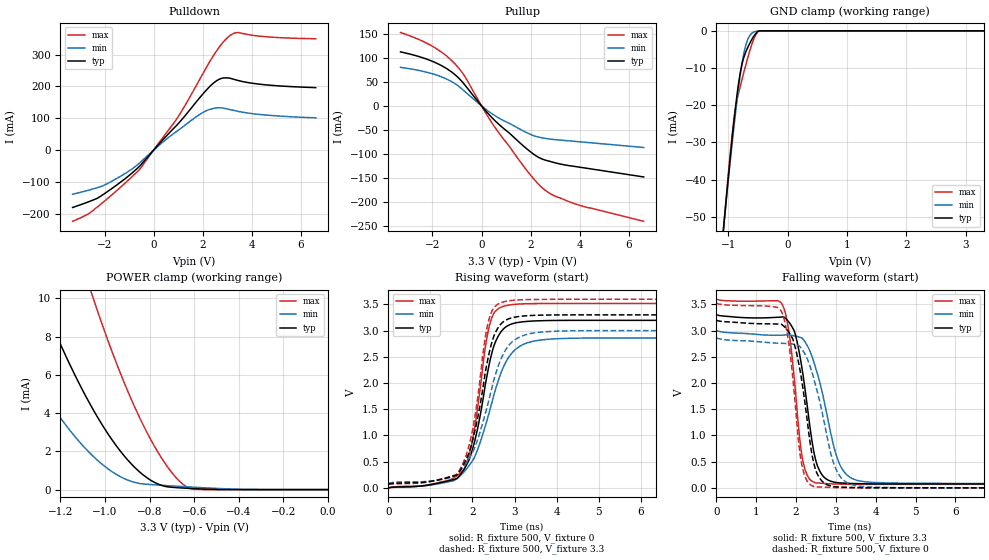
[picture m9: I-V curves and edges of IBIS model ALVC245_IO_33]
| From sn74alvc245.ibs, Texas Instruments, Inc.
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[Model]   ALVC245_IO_33
Model_type  I/O
Vinl=0.8
Vinh=2.0
Enable   Active-Low
Vref =   0
Rref =   500
Cref =   50p
Vmeas =   1.5
| variable   typ   min   max
C_comp   8.35pF   7.81pF   9.09pF
| C_pullup   10.69pF   8.03pF   12.78pF
| C_pulldown   13.57pF   8.50pF   20.76pF
| C_tri-state   8.35pF   7.81pF   9.09pF
[Temperature Range]   40   100   -40
| Ambient temperature   25   85   -40
[Voltage range]   3.3   3   3.6
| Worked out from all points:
|   slope of the pulldown table from 0 to 0.495 V, typ, clamps not added: 11.7 ohm
|   slope of the pullup table from 0 to 0.495 V, typ, clamps not added: 17.6 ohm
|   GND clamp passes 1 mA (typ) near -0.55 V on its own axis
|   POWER clamp passes 1 mA (typ) near -0.85 V on its own axis
|   rising waveform, R_fixture 500, V_fixture 0: 20-80 % time 492ps typ, 686ps min, 390ps max; typ from 0 V to 3.2 V
|   falling waveform, R_fixture 500, V_fixture 3.3: 20-80 % time 376ps typ, 552ps min, 281ps max; typ from 3.3 V to 0.073 V
|   rising waveform, R_fixture 500, V_fixture 3.3: 20-80 % time 484ps typ, 664ps min, 403ps max; typ from 0.073 V to 3.3 V
|   falling waveform, R_fixture 500, V_fixture 0: 20-80 % time 382ps typ, 537ps min, 285ps max; typ from 3.2 V to 0 V
[GND Clamp]
| ALVC245_IO_33
|   Voltage   I(typ)   I(min)   I(max)
-3.3V     -490.9mA   -462.1mA   -523.9mA
-1.08V    -53.52mA   -53.36mA   -53.54mA
-1.06V    -50.03mA   -50.1mA    -49.79mA
-965mV    -34.02mA   -35.1mA    -32.92mA
-910mV    -25.42mA   -26.89mA   -24.65mA
-865mV    -19.02mA   -20.55mA   -19.71mA
-810mV    -12.51mA   -13.51mA   -15.72mA
-765mV    -8.79mA    -8.615mA   -12.94mA
-705mV    -5.752mA   -3.933mA   -9.277mA
-575mV    -1.611mA   -356.2uA   -2.46mA
-475mV    -22.44uA   -72.78uA   -18.11uA
3.3V      121pA      1.473uA    20.6pA
[POWER Clamp]
| ALVC245_IO_33
|   Voltage   I(typ)   I(min)   I(max)
-3.3V     99.98mA    69.88mA    142.9mA
-1.515V   17.25mA    10.07mA    30.01mA
-1.39V    13.1mA     7.28mA     23.94mA
-1.295V   10.22mA    5.398mA    19.63mA
-1.175V   6.968mA    3.359mA    14.59mA
-1.055V   4.22mA     1.764mA    10.08mA
-950mV    2.303mA    801.1uA    6.651mA
-845mV    925.8uA    321uA      3.771mA
-745mV    216.5uA    225uA      1.628mA
-655mV    85.43uA    160.6uA    324.5uA
-600mV    50.05uA    123.9uA    17.12uA
-48.03fV  121pA      541.2pA    23.35pA
[Pulldown]
| ALVC245_IO_33
|   Voltage   I(typ)   I(min)   I(max)
-3.3V     -180.2mA   -138.9mA   -223.6mA
-2.675V   -163.1mA   -126.5mA   -201.3mA
-2.27V    -150.3mA   -117.4mA   -177.2mA
-1.355V   -101.2mA   -82.56mA   -117mA
-550mV    -48.67mA   -38.97mA   -58.59mA
955mV     79.19mA    59.82mA    99.87mA
1.96V     172.1mA    116.1mA    233.8mA
2.59V     219mA      132.6mA    314.7mA
3.1V      225.7mA    127.4mA    359.2mA
3.435V    218.6mA    121.6mA    369mA
4.63V     204.5mA    109.7mA    355.6mA
6.6V      196.1mA    101.2mA    349.6mA
[Pullup]
| ALVC245_IO_33
|   Voltage   I(typ)   I(min)   I(max)
-3.3V     112.1mA    79.99mA    152.2mA
-1.985V   92.16mA    66.47mA    123.3mA
-1.48V    79.23mA    57.07mA    105.8mA
-1.05V    63.39mA    45.04mA    85.45mA
-665mV    42.48mA    29.16mA    59.86mA
130mV     -7.91mA    -5.33mA    -11.38mA
615mV     -34.03mA   -22.47mA   -49.68mA
1.98V     -94.75mA   -58.81mA   -142.7mA
2.575V    -112.2mA   -67.23mA   -174.4mA
2.995V    -118.1mA   -69.95mA   -187.3mA
3.94V     -126.8mA   -74.19mA   -205.4mA
6.6V      -147.4mA   -86.26mA   -239.4mA
[Ramp]
| ALVC245_IO_33
| variable   typ   min   max
dV/dt_r   1.92/5.03E-10   1.72/6.88E-10   2.11/3.98E-10
dV/dt_f   1.94/4.01E-10   1.75/5.64E-10   2.12/2.84E-10
R_load = 500
[Rising Waveform]
| ALVC245_IO_33
R_fixture =   500
C_fixture =   0
L_fixture =   0
V_fixture =   0
V_fixture_min = 0
V_fixture_max = 0
|   Time   V(typ)   V(min)   V(max)
0s        400.7pV    3.194nV    69.15pV
1.43ns    134mV      115.4mV    143.4mV
1.8ns     356.3mV    305.9mV    346.1mV
2.02ns    792.5mV    541.5mV    996.1mV
2.31ns    1.99V      1.192V     2.703V
2.43ns    2.473V     1.533V     3.174V
2.665ns   2.962V     2.165V     3.44V
3.02ns    3.146V     2.639V     3.502V
4.8ns     3.196V     2.859V     3.519V
50ns      3.196V     2.86V      3.52V
[Falling Waveform]
| ALVC245_IO_33
R_fixture =   500
C_fixture =   0
L_fixture =   0
V_fixture =   3.3
V_fixture_min = 3
V_fixture_max = 3.6
|   Time   V(typ)   V(min)   V(max)
0s        3.3V       3V         3.6V
1.66ns    3.26V      2.913V     3.493V
1.855ns   3.127V     2.914V     2.8V
1.99ns    2.902V     2.895V     1.809V
2.165ns   2.207V     2.847V     546.2mV
2.505ns   498.4mV    2.255V     94.77mV
2.725ns   188.6mV    1.585V     82.79mV
3.115ns   93.88mV    419mV      70.85mV
3.915ns   75.69mV    104.3mV    66.63mV
50ns      73.48mV    84.08mV    66.64mV
[Rising Waveform]
| ALVC245_IO_33
R_fixture =   500
C_fixture =   0
L_fixture =   0
V_fixture =   3.3
V_fixture_min = 3
V_fixture_max = 3.6
|   Time   V(typ)   V(min)   V(max)
0s        73.48mV    84.08mV    66.64mV
1.63ns    246.6mV    259.4mV    256.5mV
1.98ns    837mV      648.4mV    1.01V
2.11ns    1.28V      894.7mV    1.636V
2.305ns   2.207V     1.416V     2.874V
2.415ns   2.636V     1.753V     3.277V
2.685ns   3.133V     2.471V     3.534V
2.99ns    3.254V     2.814V     3.58V
4.87ns    3.3V       3V         3.598V
50ns      3.3V       3V         3.6V
[Falling Waveform]
| ALVC245_IO_33
R_fixture =   500
C_fixture =   0
L_fixture =   0
V_fixture =   0
V_fixture_min = 0
V_fixture_max = 0
|   Time   V(typ)   V(min)   V(max)
0s        3.196V     2.86V      3.52V
1.64ns    3.117V     2.757V     3.357V
1.84ns    2.945V     2.75V      2.636V
2.14ns    2.065V     2.656V     465.7mV
2.375ns   750.9mV    2.268V     51.08mV
2.5ns     328.3mV    1.929V     15.85mV
2.865ns   37.21mV    680.4mV    8.122mV
3.04ns    18.11mV    298.1mV    4.51mV
3.815ns   2.126mV    16.37mV    70.65uV
50ns      865.5nV    -1.053uV   813.2nV
